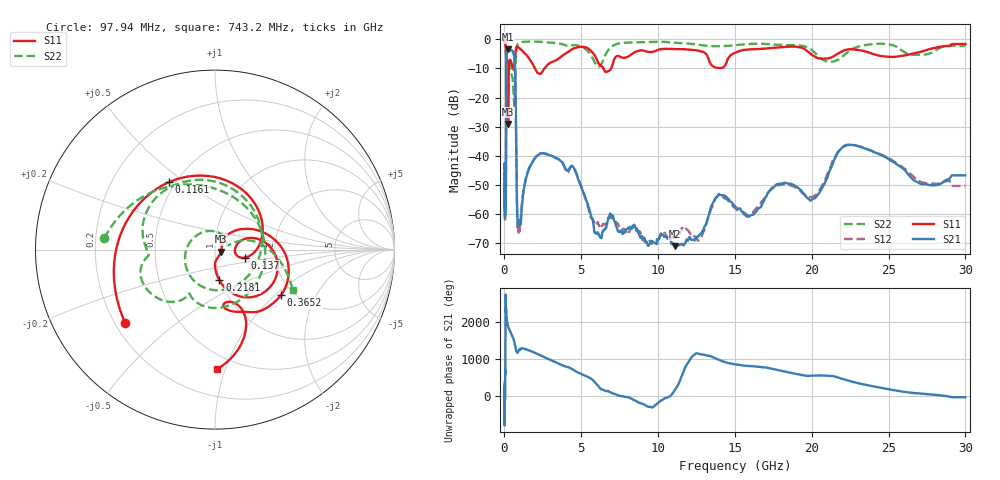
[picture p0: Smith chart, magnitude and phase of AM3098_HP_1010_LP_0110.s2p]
! Date/Time: Thu, Feb 28, 2019 8:42 AM
! Network Analyzer: Agilent Technologies E8364B Rev: A.07.50.67
! Sweep from 0.010 to 30.000 GHz, 1601 Points, Sweep Type: LOG
! Power Supply: 5.022 V, 0.002 A
# Hz S DB R 50
!freq MagS11 AngS11 MagS21 AngS21 MagS12 AngS12 MagS22 AngS22
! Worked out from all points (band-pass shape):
!   1601 points, 10 MHz to 30 GHz, reference 50 ohm
!   highest |S21| = -3.44 dB at 238.7 MHz (marker M1); lowest = -71.2 dB at 11.08 GHz (marker M2)
!   |S21| within 3 dB of the highest: 132.9 MHz to 644.9 MHz (512 MHz wide, 132 % of centre)
!   lowest |S11| = -29.1 dB at 238.7 MHz (marker M3), VSWR 1.07, Z = 53.4 - j1.16 ohm
!   |S11| at or under -10 dB: 200 MHz to 289.7 MHz (89.72 MHz wide, 36.6 % of centre); 1.993 GHz to 2.602 GHz (609.1 MHz wide, 26.5 % of centre); 6.443 GHz to 6.941 GHz (498.3 MHz wide, 7.45 % of centre)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
!   |S22| runs from -23.0 to -0.6 dB; largest |S21 - S12| = 0.0099
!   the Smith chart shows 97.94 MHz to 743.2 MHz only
!   S11 on the Smith chart (normalised r, x): 97.94 MHz: 0.24, -0.34; 116.1 MHz: 0.46, +0.44; 137 MHz: 1.39, -0.13; 218.1 MHz: 0.99, -0.35; 365.2 MHz: 1.73, -1.09; 743.2 MHz: 0.39, -0.94
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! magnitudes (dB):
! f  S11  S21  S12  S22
! 10 MHz  -0.3  -44.6  -45.6  -0.6
! 38.04 MHz  -0.4  -58.8  -60.8  -0.8
! 97.94 MHz  -3.8  -46.6  -49.1  -4.2
! 116.1 MHz  -6.8  -18.7  -18.7  -10.8
! 137 MHz  -15.3  -5.6  -5.6  -10.7
! 144.7 MHz  -19.1  -4.8  -4.8  -10.8
! 218.1 MHz  -15.3  -3.6  -3.5  -8.2
! 238.7 MHz  -29.1  -3.4  -3.4  -8.6
! 365.2 MHz  -7.0  -3.8  -3.7  -7.9
! 550.5 MHz  -9.8  -4.3  -4.2  -14.7
! 646.1 MHz  -9.6  -6.5  -6.5  -22.9
! 743.2 MHz  -3.5  -25.8  -25.8  -6.2
! 825.6 MHz  -2.4  -59.1  -61.0  -2.1
! 917.1 MHz  -2.7  -63.5  -66.0  -1.3
! 2.084 GHz  -10.9  -40.3  -40.2  -0.8
! 4.458 GHz  -3.2  -43.8  -43.8  -1.9
! 6.08 GHz  -7.8  -66.5  -62.9  -9.4
! 7.926 GHz  -6.2  -65.6  -66.3  -1.1
! 11.08 GHz  -3.3  -71.2  -68.2  -1.1
! 20.1 GHz  -5.6  -54.9  -54.1  -4.1
! 22.67 GHz  -3.4  -36.4  -36.3  -3.2
! 30 GHz  -1.6  -46.8  -50.5  -2.2
